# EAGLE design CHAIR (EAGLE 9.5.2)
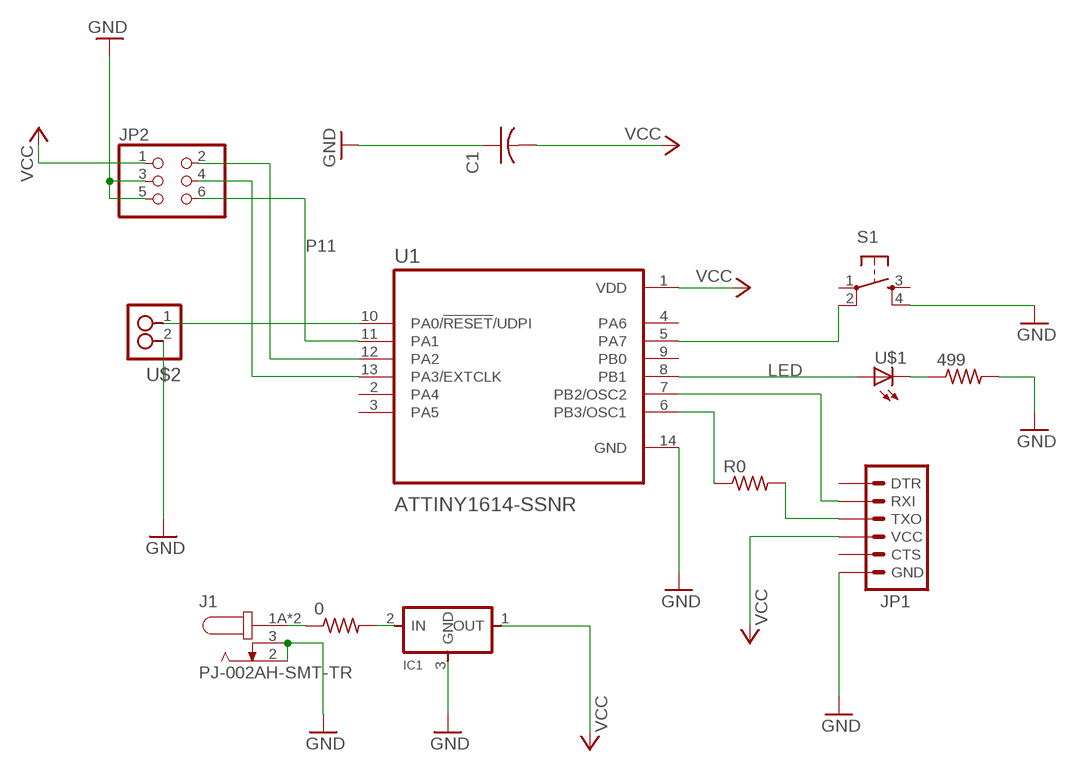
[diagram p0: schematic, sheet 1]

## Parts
0  RESISTOR1206  [1206]
499  RESISTOR1206  [1206]
C1  C-USC1206  [C1206]
IC1  REGULATORSOT23  [SOT23]
J1  PJ-002AH-SMT-TR  [CUI_PJ-002AH-SMT-TR]
JP1  FTDI_CONNECTORSMD  [1X06]
JP2  PINHD-2X3-SMD  [2X03SMD]
R0  RESISTOR1206  [1206]
S1  6MM_SWITCH6MM_SWITCH  [6MM_SWITCH]
U1  ATTINY1614-SSNR  [SOIC127P600X175-14N]
U$1  LED1206  [1206]
U$2  2_PIN_HEADERHEADER  [SMT_PINS_2]

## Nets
GND: 499.2 C1.1 IC1.3(GND) J1.2 J1.3 JP1.6(GND) JP2.3 JP2.5 S1.4(S1) U1.14(GND) U$2.2
LED: U1.8(PB1) U$1.1(A)
N$1: JP1.3(TXO) R0.2
N$2: R0.1 U1.6(PB3/OSC1)
N$3: JP1.2(RXI) U1.7(PB2/OSC2)
N$5: U1.10(PA0/!RESET!/UDPI) U$2.1
N$6: S1.2(P1) U1.5(PA7)
N$7: 0.2 IC1.2(IN)
N$8: 499.1 U$1.2(C)
N$9: JP2.2 U1.12(PA2)
N$10: JP2.4 U1.13(PA3/EXTCLK)
N$11: 0.1 J1.1A J1.1B
P11: JP2.6 U1.11(PA1)
VCC: C1.2 IC1.1(OUT) JP1.4(VCC) JP2.1 U1.1(VDD)
Unconnected: JP1.1(DTR) JP1.5(CTS) S1.1(P) S1.3(S) U1.2(PA4) U1.3(PA5) U1.4(PA6) U1.9(PB0)

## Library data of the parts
0 499 R0 = fablab:RESISTOR
C1 = rcl:C-US: CAPACITOR, American symbol; SPICEPREFIX: C
IC1 = fablab:REGULATOR
J1 = PJ-002AH-SMT-TR:PJ-002AH-SMT-TR: 2.0 mm Center Pin, 5.0 A, Right Angle, Surface Mount (SMT), Dc Power Jack Connector; AVAILABILITY: Unavailable; CUI_PURCHASE_URL: https://www.cuidevices.com/product/interconnect/connectors/dc-power-connectors/jacks/pj-002ah-smt-tr?utm_source=snapeda.com&utm_medium=referral&utm_campaign=snapedaBOM; DESCRIPTION: 2.0 x 6.5 mm, 5.0 A, Horizontal, Surface Mount _SMT_, Dc Power Jack Connector; MF: CUI Devices; MP: PJ-002AH-SMT-TR; PACKAGE: None; PRICE: None
JP1 = fablab:FTDI_CONNECTOR: FTDI connector smd
JP2 = fablab:PINHD-2X3-SMD: PIN HEADER
S1 = fablab:6MM_SWITCH: OMRON SWITCH
U1 = ATTINY1614-SSNR:ATTINY1614-SSNR: 20MHz, SOIC, 85C, Green, 14 SOIC .150in T/R; AVAILABILITY: Unavailable; DESCRIPTION: AVR tinyAVR™ 1 Microcontroller IC 8-Bit 20MHz 16KB _16K x 8_ FLASH 14-SOIC; MF: Microchip; MP: ATTINY1614-SSNR; PACKAGE: SO-14 Microchip; PRICE: None
U$1 = fablab:LED
U$2 = fablab:2_PIN_HEADER: 2 SMT pin pads

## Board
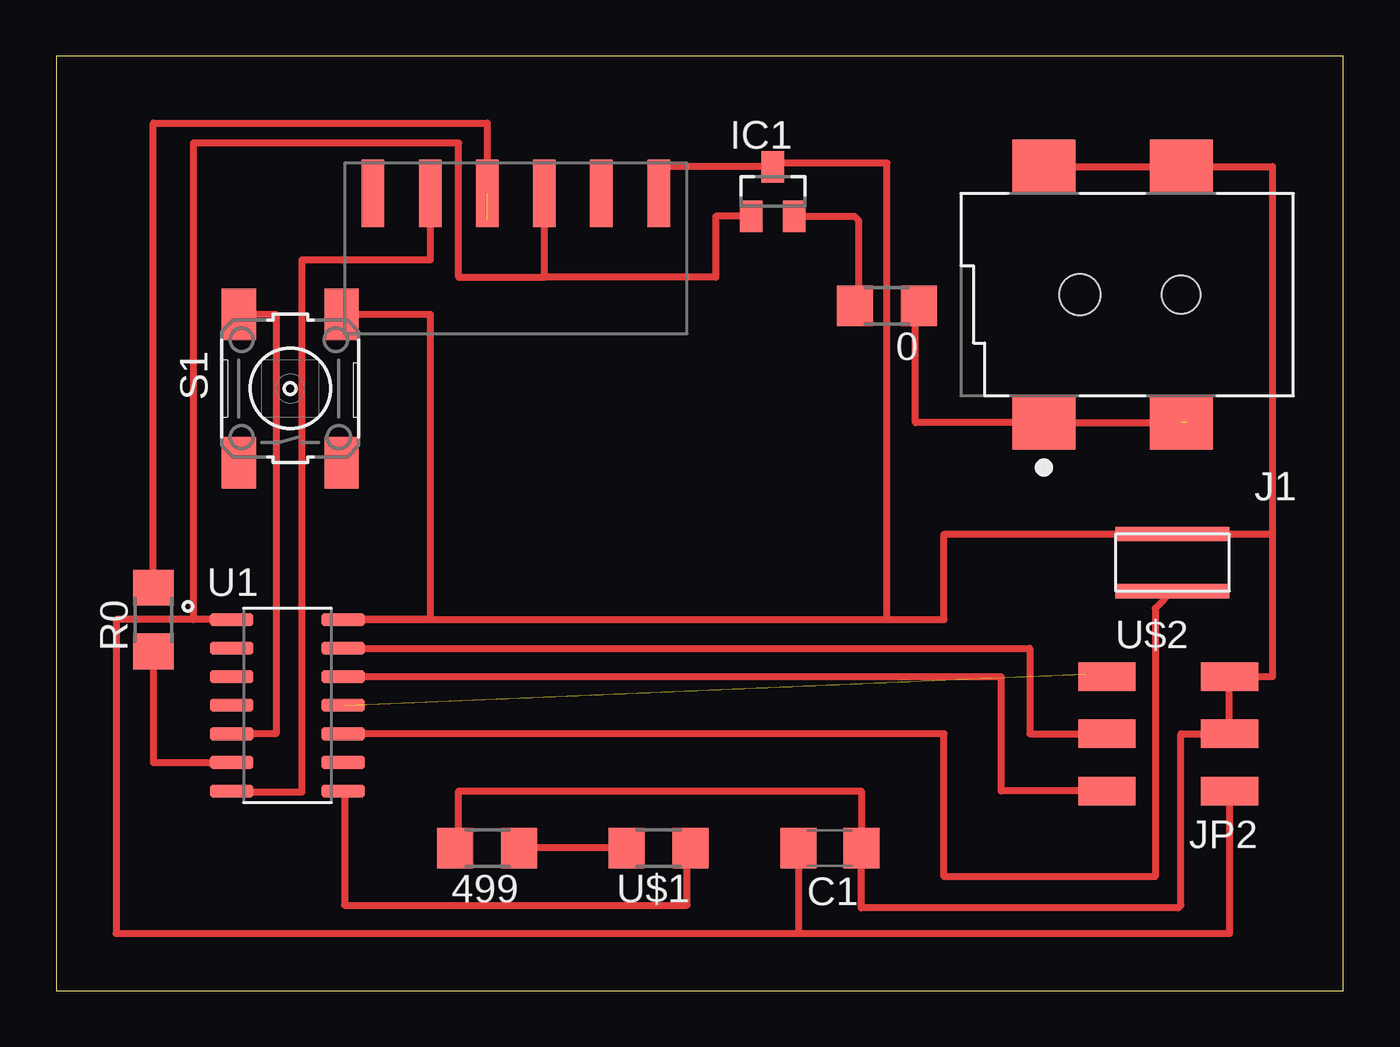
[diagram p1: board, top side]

Size 57.26 x 41.58 mm. Coordinates in mm from the lower left corner, seen from the top.
Outline: 0,0 57.26,0 57.26,41.58 0,41.58 0,0
Copper layers (1*16): Top 0.035mm / dielectric 1.5mm / Bottom 0.035mm
Design rules "default": minimum track width 6mil, minimum drill 0.35mm, track to track 6mil, track to pad 6mil, pad to pad 6mil, via to via 6mil, smd to smd 6mil, copper to edge 40mil, drill to drill 6mil, minimum pad ring 10mil, minimum via ring 8mil, stop-mask expansion 4mil, vias tented up to drill 0mil, thermal gap 10mil

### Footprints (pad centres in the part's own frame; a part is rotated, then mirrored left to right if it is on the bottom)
1206 = smd 1.6 x 1.803: 1 -1.422,0; 2 1.422,0
C1206 = smd 1.6 x 1.8: 1 -1.4,0; 2 1.4,0
SOT23 = smd 1 x 1.4: 1 -0.95,-1.1; 2 0.95,-1.1; 3 0,1.1
CUI_PJ-002AH-SMT-TR = smd 2.8 x 2.4: 1A 0,0; 1B -6.1,0; 2 -6.1,-11.4; 3 0,-11.4 | hole 1.7: -6.1,-5.7 | hole 1.8: -1.6,-5.7
1X06 = smd 1 x 3: 1 -6.35,5; 2 -3.81,5; 3 -1.27,5; 4 1.27,5; 5 3.81,5; 6 6.35,5
2X03SMD = smd 2.54 x 1.27: 1 -2.54,2.54; 2 2.92,2.54; 3 -2.54,0; 4 2.92,0; 5 -2.54,-2.54; 6 2.92,-2.54
6MM_SWITCH = smd 2.286 x 1.524: 1 -3.302,2.286; 2 3.302,2.286; 3 -3.302,-2.286; 4 3.302,-2.286
SOIC127P600X175-14N = smd 1.95 x 0.59: 1 -2.48,3.81; 2 -2.48,2.54; 3 -2.48,1.27; 4 -2.48,0; 5 -2.48,-1.27; 6 -2.48,-2.54; 7 -2.48,-3.81; 8 2.48,-3.81; 9 2.48,-2.54; 10 2.48,-1.27; 11 2.48,0; 12 2.48,1.27; 13 2.48,2.54; 14 2.48,3.81
SMT_PINS_2 = smd 5.08 x 0.635: 1 0,0; 2 0,2.54

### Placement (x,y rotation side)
0  36.96,30.48 180 top
499  19.18,6.35 180 top
C1  34.42,6.35 180 top
IC1  31.88,35.56 0 top
J1  43.94,25.27 180 top
JP1  20.45,30.48 0 top
JP2  49.66,11.43 180 top
R0  4.32,16.51 90 top
S1  10.41,26.8 90 top
U1  10.29,12.7 0 top
U$1  26.8,6.35 180 top
U$2  49.66,17.78 0 top

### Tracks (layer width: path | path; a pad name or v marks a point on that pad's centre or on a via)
GND
  Top 0.305: 17.91,6.2 499.2 17.91,6.5 17.91,8.89 35.82,8.89 C1.1 35.81,3.68 49.91,3.68 50.04,3.81 50.04,11.43 JP2.3 JP2.5 54.1,13.97 54.1,20.32 | 54.1,20.32 U$2.2 39.5,20.32 39.5,16.51 U1.14 | JP1.6 26.8,36.66 IC1.3 32.05,36.83 36.96,36.83 36.96,16.51 U1.14 | S1.4 16.64,30.1 16.64,16.51 U1.14 | 54.1,20.32 54.1,36.67 J1.2 J1.3
LED
  Top 0.305: U$1.1 28.07,6.5 28.07,3.81 12.83,3.81 12.83,8.83 U1.8
N$1  (1 unrouted)
  Top 0.305: 19.18,34.29 19.18,38.61 4.32,38.61 R0.2
N$2
  Top 0.305: 4.17,15.24 R0.1 4.32,10.16 U1.6
N$3
  Top 0.305: U1.7 7.75,8.83 10.92,8.83 10.92,32.51 16.64,32.51 JP1.2
N$5
  Top 0.305: U$2.1 48.89,17.02 48.89,5.08 39.5,5.08 39.5,11.43 U1.10
N$6
  Top 0.305: S1.2 9.78,30.1 9.78,11.43 U1.5
N$7
  Top 0.305: IC1.2 35.52,34.46 35.69,34.29 35.69,30.63 0.2
N$8
  Top 0.305: U$1.2 499.1 20.45,6.2
N$9
  Top 0.305: JP2.2 42.04,8.89 42.04,13.97 U1.12
N$10
  Top 0.305: U1.13 43.31,15.24 43.31,11.43 JP2.4
N$11  (1 unrouted)
  Top 0.305: 0.1 38.23,30.63 38.23,25.27 J1.1A 50.29,25.27
P11  (1 unrouted)
  Top 0.305: 47.12,14.35 JP2.6 46.74,14.1 45.85,14.1
VCC
  Top 0.305: U1.1 7.75,16.57 | 30.61,34.14 IC1.1 29.34,34.46 29.34,31.75 21.72,31.75 | 21.72,31.75 JP1.4 | U1.1 6.92,16.51 | 21.72,31.75 17.91,31.75 17.91,37.72 6.1,37.72 6.1,16.51 | C1.2 33.02,2.54 | 33.02,2.54 2.67,2.54 2.67,16.51 6.1,16.51 | U1.1 6.1,16.51 | JP2.1 52.2,2.54 33.02,2.54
